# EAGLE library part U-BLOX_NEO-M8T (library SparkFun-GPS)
u-blox NEO-M8T The NEO-M8T and LEA-M8T concurrent GNSS modules deliver high integrity, precision timing in demanding applicationsworld-wide. Support for BeiDou, GLONASS and Galileo constellations enables compliance with national requirements. Enhanced sensitivity and concurrent constellation reception extend coverage and integrity to challenging signal environments. Survey-in and fixed-position navigation reduce timing jitter, even at low signal levels, and enable synchronization to be maintained with as few as one single satellite in view. Support for low duty cycle operation reduces power consumption for battery-powered applications. u-blox timing products include timing integrity measures with Receiver Autonomous Integrity Monitoring (RAIM) and continuous phase uncertainty estimation. They feature high dynamic range radios with both analog and digital interference mitigation, supporting applications in wireless communications equipment. The M8T timing modules are delivered in u-blox’s established LEA and NEO form-factors with standard pin-out, allowing ready migration from previous product generations. u-blox timing products can make use of u-blox AssistNow or industry-standard aiding data. This reduces the time-to-firstfix and delivers exceptional acquisition sensitivity, even on first installation before precise location, time or frequency are known.
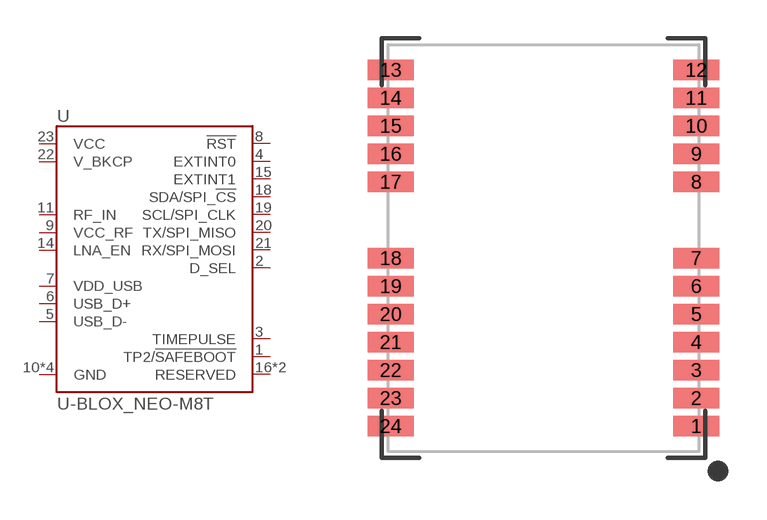
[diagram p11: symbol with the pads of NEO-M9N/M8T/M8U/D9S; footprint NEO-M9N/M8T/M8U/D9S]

Designator prefix -

## U-BLOX_NEO-M8T (PROD_ID: IC-14839)  [NEO-M9N/M8T/M8U/D9S]
1  TP2/!SAFEBOOT!
2  D_SEL
3  TIMEPULSE
4  EXTINT0
5  USB_D-
6  USB_D+
7  VDD_USB
8  !RST
9  VCC_RF
10  GND
11  RF_IN
12  GND
13  GND
14  LNA_EN
15  EXTINT1
16  RESERVED  nc
17  RESERVED  nc
18  SDA/SPI_!CS!
19  SCL/SPI_CLK
20  TX/SPI_MISO
21  RX/SPI_MOSI
22  V_BKCP
23  VCC
24  GND

## Footprint NEO-M9N/M8T/M8U/D9S (pad centres in mm)
u-blox NEO-M9N/M8T/M8U/D9S Module Mechanical Specifications Overall: 12.2mm x 16.0mm Pad Pitch: 1.1mm Pad Width: .8mm Pad Length: .9mm Number of Pins: 24
smd 1.8 x 0.8: 1 6,-7; 2 6,-5.9; 3 6,-4.8; 4 6,-3.7; 5 6,-2.6; 6 6,-1.5; 7 6,-0.4; 8 6,2.6; 9 6,3.7; 10 6,4.8; 11 6,5.9; 12 6,7; 13 -6,7; 14 -6,5.9; 15 -6,4.8; 16 -6,3.7; 17 -6,2.6; 18 -6,-0.4; 19 -6,-1.5; 20 -6,-2.6; 21 -6,-3.7; 22 -6,-4.8; 23 -6,-5.9; 24 -6,-7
